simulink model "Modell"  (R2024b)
settings: Solver=FixedStepAuto  StartTime=0.0  StopTime=inf  FixedStep=0.01  RelTol=1e-3  EnableMultiTasking=on
libraries: arduinolib x2, simulink x1, simulink_extras x1

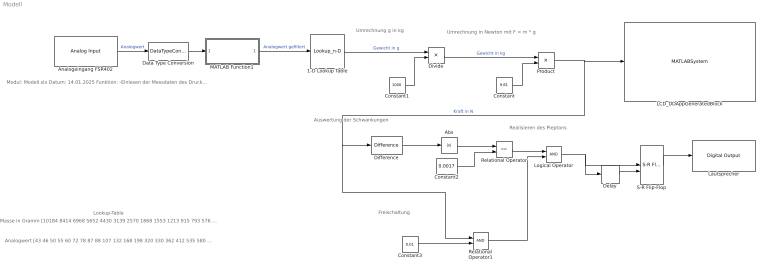
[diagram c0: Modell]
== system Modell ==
  note: Modul: Modell.slx Datum: 14.01.2025 Funktion: -Einlesen der Messdaten des Drucksensors FSR402 -Umrechnung der Analogwerte in g, kg und Newton -Ausgabe der Kraft in Newton mit einem LCD -Bestätigung der Messung durch Piepton Implementierung: Simulink Toolbox: Simulink Support Package for Arduino Hardware Simulink Extras Autor: Jan Steffens, Lukas Berkemeier Letzte Änderung: 06.02.2025
  note: Lookup-Table
  note: Umrechnung in Newton mit F = m * g
  note: Umrechnung g in kg
  note: Realisieren des Pieptons
  note: Freischaltung
  note: Auswertung der Schwankungen
  note: Masse in Gramm [10184 8414 6968 5652 4430 3139 2570 1868 1553 1213 915 793 576 338 261 218 160 130 118 101 70 54 50 46 42 0]
  note: Analogwert [43 46 50 55 60 72 78 87 88 107 132 168 198 320 330 362 412 535 580 627 790 875 925 950 970 1005]
  1-D Lookup Table : Lookup_n-D  NumberOfTableDimensions=1  BreakpointsForDimension1=[43 46 50 55 60 72 78 87 88 99 132 168 198 320 330 362 412 535 580 627 790 875 925 950 995 1005]  BreakpointsForDimension1DataTypeStr=Inherit: Inherit from 'Breakpoint data'  Table=[10184 8414 6968 5652 4430 3139 2570 1868 1553 1365 915 793 576 338 261 218 160 130 118 101 70 54 50 46 42 0]  TableDataTypeStr=uint16  ExtrapMethod=Clip  InternalRulePriority=Speed  RndMeth=Simplest
  Abs : Abs
  Analogeingang FSR402 : arduinolib/Analog Input  pinNumber=0  ReadResultsOnly=off  ConversionTriggerSource=Software  ExternalTriggerType=uint32( 0 )  OutputDataType=uint16  EnableConversionCompleteNotify=off  EnableOuputStatus=off  SampleTime=0.01  blockPlatform=arduino
  Constant : Constant  Value=9.81
  Constant1 : Constant  Value=1000
  Constant2 : Constant  Value=0.0017
  Constant3 : Constant  Value=0.01
  Data Type Conversion : DataTypeConversion  OutDataTypeStr=double
  Delay : Delay  DelayLength=5  InitialCondition=0
  Difference : simulink/Discrete/Difference  ICPrevInput=0.0  OutMin=[]  OutMax=[]  OutDataType=fixdt(1, 16)  OutScaling=2^-10  DoSatur=off
  Divide : Product  Inputs=*/
  LCD_DDAppGeneratedBlock : MATLABSystem  System=LCD  SampleTime=-1
  Lautsprecher : arduinolib/Digital Output  pinNumber=3  Direction=output  blockPlatform=arduino
  Logical Operator : Logic  AllPortsSameDT=off  OutDataTypeStr=boolean
  MATLAB Function1 : MATLAB Function  TreatAsAtomicUnit=on
  Product : Product  OutDataTypeStr=double
  Relational Operator : RelationalOperator  Operator=<=  OutDataTypeStr=boolean  RndMeth=Simplest
  Relational Operator1 : RelationalOperator  OutDataTypeStr=boolean  RndMeth=Simplest
  S-R Flip-Flop : simulink_extras/Flip Flops/S-R Flip-Flop  initial_condition=0
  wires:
  Constant/1 -> Product/2
  Delay/1 -> S-R Flip-Flop/2
  Logical Operator/1 -> S-R Flip-Flop/1, Delay/1
  S-R Flip-Flop/1 -> Lautsprecher/1
  MATLAB Function1/1(y) -> 1-D Lookup Table/1  "Analogwert gefiltert"
  Analogeingang FSR402/1 -> Data Type Conversion/1  "Analogwert"
  Data Type Conversion/1 -> MATLAB Function1/1(u)
  Product/1 -> LCD_DDAppGeneratedBlock/1, Relational Operator1/1, Difference/1  "Kraft in N"
  Relational Operator1/1 -> Logical Operator/2
  Relational Operator/1 -> Logical Operator/1
  Constant3/1 -> Relational Operator1/2
  Difference/1 -> Abs/1
  Abs/1 -> Relational Operator/1
  Constant2/1 -> Relational Operator/2
  1-D Lookup Table/1 -> Divide/1  "Gewicht in g"
  Constant1/1 -> Divide/2
  Divide/1 -> Product/1  "Gewicht in kg"

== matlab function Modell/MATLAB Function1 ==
%**************************************************************************
%        Hochschule Hamm-Lippstadt                                        *
%**************************************************************************
% Modul	          : Modell.slx                                            *
%                                                                         *
% Datum           : 14.01.2025                                            *
%                                                                         *
% Funktion        : Tiefpassfilter                                        *
%                                                                         *
% Implementation  : MATLAB R2024b                                         *
%                                                                         *                                                                     
% Author          : Jan Steffens, Lukas Berkemeier                        *
%                                                                         *                                                              
% Letzte Änderung : 06. Februar 2025                                      *
%                                                                         *
%**************************************************************************


function y = lowpass_filter_25(u)
% Tiefpassfilter mit 25 Elementen für Simulink MATLAB Function Block
% Eingabe:  u - skalare Eingabe (double)
% Ausgabe:  y - gefilterte Ausgabe (double)

persistent buffer sum_buffer;
if isempty(buffer)
    buffer = zeros(1,40); % Initialisiere den Puffer mit Nullen
    sum_buffer = 0;
end

% Ältestes Element entfernen und neues hinzufügen
sum_buffer = sum_buffer - buffer(1) + u;
buffer = [buffer(2:end), u];

% Berechne den gleitenden Durchschnitt
y = sum_buffer / 40;
end
